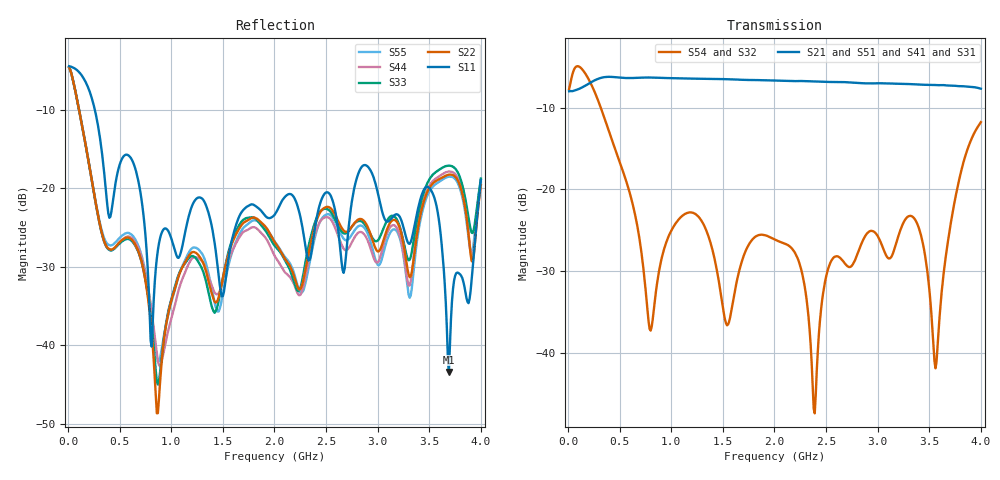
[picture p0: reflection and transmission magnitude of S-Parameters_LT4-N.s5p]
! MTS Systemtechnik GmbH
! S-Parameters
! Model: LT4-588P-4G
! Rohde & Schwarz ZVB8 2Ports - Version 3.20 - 1145.1010k08 SN: 100119
! Converted & adapted with MATLAB
!		|  MTS  |
!		|  |--o OUT 4 (Port 5)
!		|  |--o OUT 3 (Port 4)
! C (Port 1) o--| LT4-588P-4G |
!		|  |--o OUT 2 (Port 3)
!		|  |--o OUT 1 (Port 2)
! S5P File: Measurements:
! <S11,S12,S13,S14,S15>,
! <S21,S22,S23,S24,S25>,
! <S31,S32,S33,S34,S35>,
! <S41,S42,S43,S44,S45>,
! <S51,S52,S53,S54,S55>:
# HZ  S  DB  R  50.00
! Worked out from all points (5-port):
!   400 points, 10 MHz to 4 GHz, reference 50 ohm
!   strongest paths, dB at 10 MHz, 1.01 GHz, 2.01 GHz, 3.01 GHz, 4 GHz:
!     S21: -8.0, -6.4, -6.7, -7.0, -7.7
!     S51: -8.0, -6.4, -6.7, -7.0, -7.8
!     S41: -8.0, -6.4, -6.7, -7.0, -7.8
!     S31: -8.0, -6.4, -6.7, -7.1, -7.8
!     S54: -7.7, -24.8, -26.2, -25.9, -11.8
!     S32: -7.7, -24.8, -26.2, -25.9, -11.8
!   lowest |S11| = -43.4 dB at 3.69 GHz (marker M1), VSWR 1.01, Z = 50.7 - j0.195 ohm
!   |S11| at or under -10 dB: 258.8 MHz to end of sweep
